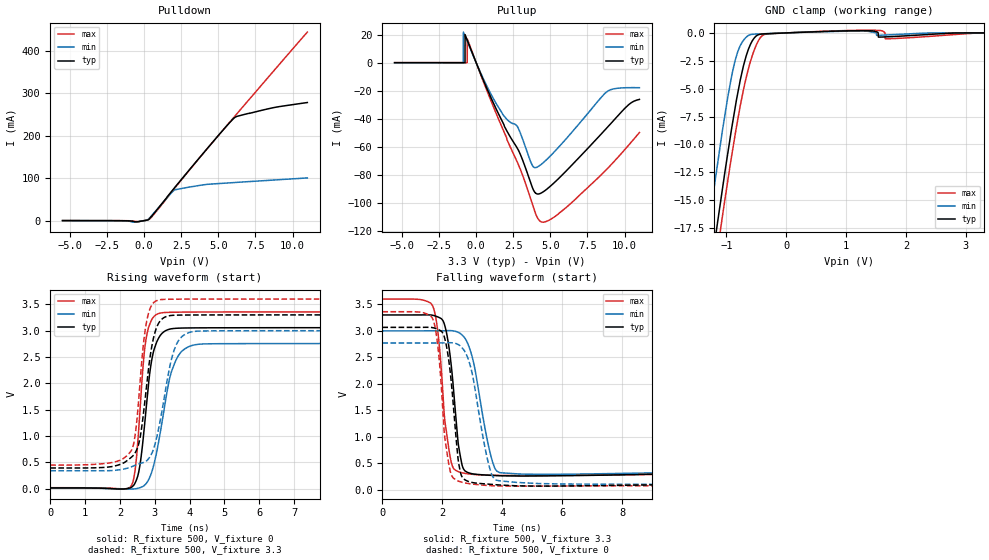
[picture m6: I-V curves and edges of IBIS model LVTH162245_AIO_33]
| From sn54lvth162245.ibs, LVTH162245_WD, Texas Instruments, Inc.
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[Model]   LVTH162245_AIO_33
Model_type  I/O
Vinl = 0.8
Vinh = 2.0
Enable   Active-Low
Vref =   0
Rref =   500
Cref =   50p
Vmeas =   1.5
| variable   typ   min   max
C_comp   10.0pF   NA   NA
| C_pullup   1.31pF   0.65pF   2.35pF
| C_pulldown   4.19pF   3.26pF   4.80pF
| C_tri-state   5.24pF   4.05pF   6.34pF
[Temperature Range]   40   -40   100
| Ambient temperature   25   -40   85
[Voltage range]   3.3   3   3.6
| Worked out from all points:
|   slope of the pulldown table from 0 to 0.495 V, typ, clamps not added: 50 ohm
|   slope of the pullup table from 0 to 0.495 V, typ, clamps not added: 38.7 ohm
|   GND clamp passes 1 mA (typ) near -0.60 V on its own axis
|   rising waveform, R_fixture 500, V_fixture 0: 20-80 % time 303ps typ, 463ps min, 229ps max; typ from 0.016 V to 3.06 V
|   falling waveform, R_fixture 500, V_fixture 3.3: 20-80 % time 300ps typ, 511ps min, 290ps max; typ from 3.3 V to 0.383 V
|   rising waveform, R_fixture 500, V_fixture 3.3: 20-80 % time 340ps typ, 466ps min, 268ps max; typ from 0.395 V to 3.3 V
|   falling waveform, R_fixture 500, V_fixture 0: 20-80 % time 305ps typ, 525ps min, 306ps max; typ from 3.07 V to 0.02 V
[GND Clamp]
| LVTH162245_AIO_33
|   Voltage   I(typ)   I(min)   I(max)
-5.5V     -196.5mA   -192.9mA   -198.4mA
-1.305V   -22.96mA   -17.75mA   -25.42mA
-1.15V    -17.06mA   -11.82mA   -19.53mA
-1.07V    -14.12mA   -8.863mA   -16.57mA
-845mV    -6.415mA   -2.299mA   -8.821mA
-670mV    -2.066mA   -388.5uA   -4.024mA
-500mV    -269uA     -104.7uA   -1.076mA
-275mV    -63.13uA   -55.67uA   -75.86uA
1.35V     194.4uA    153.1uA    238.8uA
1.54V     -379uA     -218.8uA   223.4uA
1.655V    -359.4uA   -190.5uA   -529.7uA
3.3V      31.16pA    26.13pA    -1.135uA
[Pulldown]
| LVTH162245_AIO_33
|   Voltage   I(typ)   I(min)   I(max)
-5.5V     -24.1uA    -149.1uA   -89.1uA
-1.295V   -487.6uA   -582.2uA   -262.3uA
-665mV    -2.521mA   -3.81mA    -1.534mA
210mV     1.186mA    1.186mA    1.191mA
380mV     5.162mA    6.683mA    4.042mA
1.685V    61.48mA    59.4mA     60.02mA
2.07V     78.09mA    72.13mA    76.77mA
4.14V     164.8mA    84.74mA    164.5mA
5.545V    221.9mA    88.25mA    222.3mA
6.12V     242.7mA    89.58mA    245.8mA
8.685V    265.4mA    95.27mA    350.1mA
11V       277.7mA    100.3mA    443.4mA
[Pullup]
| LVTH162245_AIO_33
|   Voltage   I(typ)   I(min)   I(max)
-5.5V     74.95uA    40.9uA     129.2uA
-870mV    62.27uA    33.41uA    109.8uA
-865mV    62.03uA    21.91mA    109.8uA
-755mV    43.05uA    19.08mA    100.6uA
-750mV    20.1mA     18.95mA    99.32uA
-605mV    16.19mA    15.24mA    66.72uA
-600mV    16.05mA    15.11mA    17.08mA
2.795V    -61.44mA   -45.84mA   -71.53mA
3.81V     -89.66mA   -73.7mA    -101.5mA
4.44V     -92.59mA   -71.99mA   -113.7mA
8.805V    -46.47mA   -20.69mA   -75.93mA
11V       -26.14mA   -17.79mA   -49.79mA
[Ramp]
| LVTH162245_AIO_33
| variable   typ   min   max
dV/dt_r   1.84/3.08E-10   1.66/4.75E-10   2.02/2.36E-10
dV/dt_f   1.83/3.13E-10   1.63/5.23E-10   2.00/3.17E-10
R_load = 500
[Rising Waveform]
| LVTH162245_AIO_33
R_fixture =   500
C_fixture =   0
L_fixture =   0
V_fixture =   0
V_fixture_min = 0
V_fixture_max = 0
|   Time   V(typ)   V(min)   V(max)
0s        15.79mV    9.907mV    20.88mV
2.31ns    20.21mV    -5.687mV   41.24mV
2.435ns   111.1mV    -525.7uV   357mV
2.55ns    357.4mV    16.17mV    1.239V
2.76ns    1.579V     106.4mV    2.883V
2.95ns    2.568V     401.1mV    3.248V
3.255ns   2.976V     1.454V     3.343V
3.66ns    3.047V     2.507V     3.351V
4.38ns    3.054V     2.748V     3.354V
50ns      3.058V     2.757V     3.357V
[Falling Waveform]
| LVTH162245_AIO_33
R_fixture =   500
C_fixture =   0
L_fixture =   0
V_fixture =   3.3
V_fixture_min = 3
V_fixture_max = 3.6
|   Time   V(typ)   V(min)   V(max)
0s        3.3V       3V         3.6V
1.66ns    3.296V     3.001V     3.489V
1.855ns   3.262V     3.001V     2.968V
2.025ns   3.188V     3.002V     1.785V
2.325ns   2.211V     3.003V     470.7mV
2.55ns    804.6mV    2.968V     340.5mV
2.895ns   318.4mV    2.697V     299.3mV
3.635ns   274mV      613.2mV    273.4mV
4.015ns   264.6mV    319.1mV    270.9mV
50ns      382.6mV    337.5mV    431.9mV
[Rising Waveform]
| LVTH162245_AIO_33
R_fixture =   500
C_fixture =   0
L_fixture =   0
V_fixture =   3.3
V_fixture_min = 3
V_fixture_max = 3.6
|   Time   V(typ)   V(min)   V(max)
0s        394.6mV    342.7mV    449mV
2.32ns    594.1mV    414.7mV    717.6mV
2.44ns    685.2mV    447mV      1.039V
2.56ns    912.7mV    475.3mV    1.876V
2.78ns    2.043V     539.9mV    3.222V
2.965ns   2.868V     756.9mV    3.53V
3.195ns   3.214V     1.437V     3.591V
3.605ns   3.295V     2.716V     3.598V
4.225ns   3.298V     2.992V     3.6V
50ns      3.3V       3V         3.6V
[Falling Waveform]
| LVTH162245_AIO_33
R_fixture =   500
C_fixture =   0
L_fixture =   0
V_fixture =   0
V_fixture_min = 0
V_fixture_max = 0
|   Time   V(typ)   V(min)   V(max)
0s        3.066V     2.77V      3.361V
1.65ns    3.063V     2.771V     3.257V
1.84ns    3.031V     2.772V     2.77V
2.01ns    2.964V     2.772V     1.581V
2.26ns    2.25V      2.776V     368.2mV
2.59ns    373.5mV    2.719V     154.5mV
3.06ns    132.3mV    2.013V     105.3mV
3.655ns   101.9mV    284.3mV    77.79mV
4.495ns   75.24mV    139.2mV    68.94mV
50ns      20.02mV    12.37mV    23.58mV
